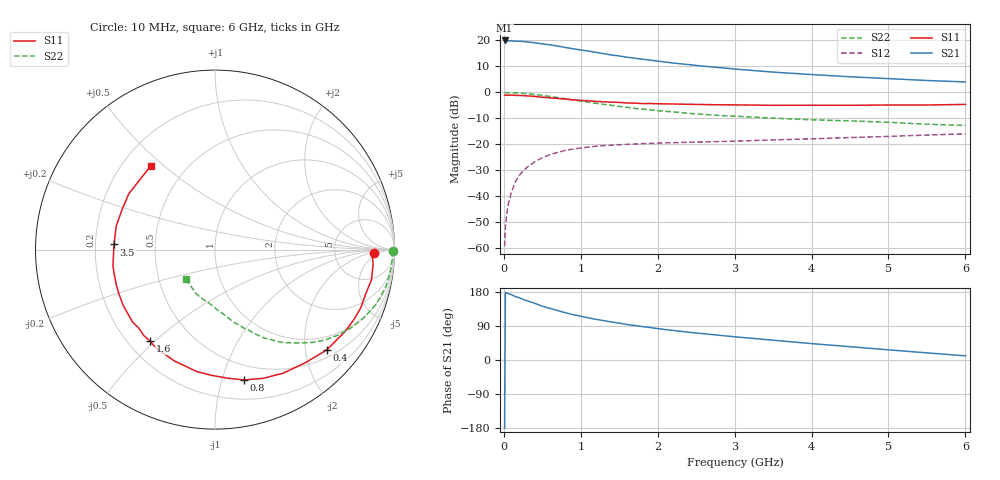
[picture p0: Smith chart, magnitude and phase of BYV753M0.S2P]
! SIEMENS Small Signal Semiconductors
! BFY420
! Si NPN RF SIEGET Grounded Emitter Transistor in MICRO-X
! VCE = 0.75 V  IC = 3 mA
! Common Emitter S-Parameters:  October  1996
# GHz  S  MA  R  50
!  f  S11  S21  S12  S22
! GHz  MAG  ANG  MAG  ANG  MAG  ANG  MAG  ANG
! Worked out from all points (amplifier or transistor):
!   36 points, 10 MHz to 6 GHz, reference 50 ohm
!   highest |S21| = 20.0 dB at 10 MHz (marker M1)
!   |S21| within 3 dB of that: start of sweep to 859.5 MHz
!   unconditionally stable (mu >= 1): 3.496 GHz to end of sweep
!   at 250 MHz: K = 0.08, MSG = 24.9 dB, |S12| = -30.3 dB
!   at 1.4 GHz: K = 0.41, MSG = 17.4 dB, |S12| = -20.3 dB
!   at 6 GHz: K = 1.23, MAG = 7.1 dB, |S12| = -15.9 dB
!   S11 on the Smith chart (normalised r, x): 10 MHz: 16, -3; 400 MHz: 0.66, -2.46; 800 MHz: 0.36, -1.18; 1.6 GHz: 0.29, -0.48; 3.5 GHz: 0.28, +0.02; 6 GHz: 0.32, +0.45
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0.01  0.8856 -1.3  9.982 -179.8  0.0011 93.3  0.9917 -0.5
0.02  0.8776 -2.3  9.915 178.2  0.0026 97.6  0.9876 -1.2
0.05  0.8849 -5.4  9.772 175.5  0.0063 85.3  0.9894 -3.1
0.1  0.8879 -11.0  9.821 172.4  0.0123 84.2  0.9852 -6.4
0.15  0.8756 -16.0  9.669 167.4  0.019 79.9  0.9796 -9.7
0.25  0.8666 -26.7  9.556 160.1  0.0307 74.5  0.9586 -15.9
0.3  0.8573 -31.9  9.373 156.2  0.0362 72.0  0.9466 -18.9
0.4  0.8368 -41.9  9.002 149.8  0.0462 65.9  0.9125 -24.6
0.5  0.8063 -51.5  8.568 142.0  0.0553 60.9  0.8748 -29.9
0.6  0.7864 -61.1  8.213 136.2  0.0637 56.4  0.8346 -34.8
0.8  0.7437 -77.5  7.325 124.8  0.0765 48.1  0.7532 -43.3
0.9  0.72 -84.3  6.896 119.7  0.0811 45.0  0.715 -46.6
1.1  0.6873 -98.4  6.236 111.2  0.0889 39.4  0.6478 -53.2
1.4  0.6474 -115.2  5.243 100.2  0.0964 32.8  0.5649 -60.8
1.6  0.6256 -125.4  4.754 93.8  0.1002 29.7  0.5149 -65.0
2  0.6046 -142.4  3.998 82.8  0.1058 25.2  0.4442 -71.8
2.2  0.5987 -148.6  3.67 78.0  0.1077 23.3  0.4222 -74.9
2.8  0.5776 -166.2  2.998 65.2  0.1133 20.0  0.3589 -83.0
3.5  0.5636 177.1  2.457 52.2  0.1217 17.5  0.3196 -91.2
4.5  0.5638 156.4  1.999 35.1  0.1351 13.8  0.2828 -104.6
5.5  0.5722 136.7  1.693 18.8  0.1511 9.7  0.2438 -123.4
6  0.5876 127.7  1.59 11.0  0.1595 7.2  0.2313 -134.9
